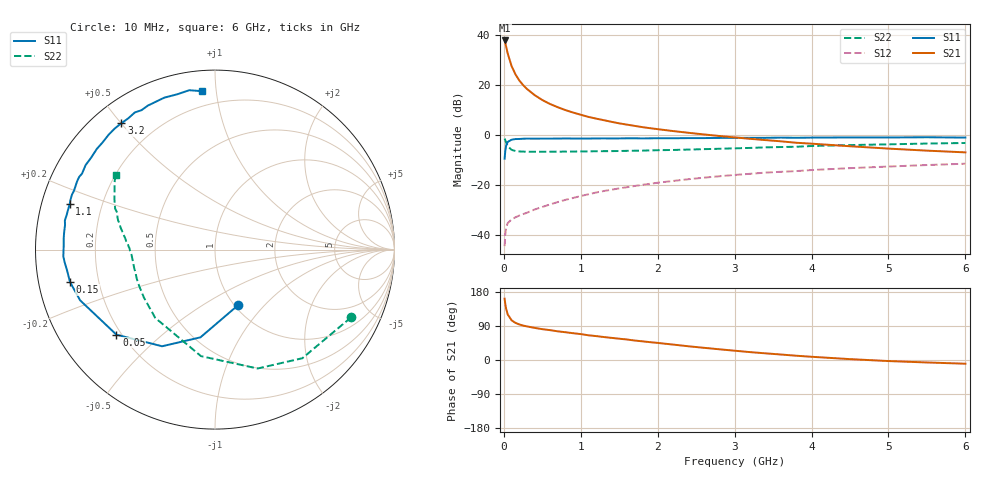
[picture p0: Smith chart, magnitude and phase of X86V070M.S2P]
! SIEMENS Small Signal Semiconductors
! BFP136W
! Si NPN RF Bipolar Junction Transistor in SOT343
! VCE = 6 V  IC = 70 mA
! Common Emitter S-Parameters:  September  1994
# GHz  S  MA  R  50
!  f  S11  S21  S12  S22
! GHz  MAG  ANG  MAG  ANG  MAG  ANG  MAG  ANG
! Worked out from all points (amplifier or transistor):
!   40 points, 10 MHz to 6 GHz, reference 50 ohm
!   highest |S21| = 37.8 dB at 10 MHz (marker M1)
!   |S21| within 3 dB of that: start of sweep to 34.05 MHz
!   unconditionally stable (mu >= 1): 612.6 MHz to 2.891 GHz
!   at 200 MHz: K = 0.59, MSG = 27.0 dB, |S12| = -32.2 dB
!   at 1.5 GHz: K = 1.10, MAG = 11.0 dB, |S12| = -21.4 dB
!   at 6 GHz: K = 0.95, MSG = 2.3 dB, |S12| = -11.5 dB
!   S11 on the Smith chart (normalised r, x): 10 MHz: 1.04, -0.72; 50 MHz: 0.18, -0.36; 150 MHz: 0.10, -0.11; 1.1 GHz: 0.08, +0.15; 3.2 GHz: 0.08, +0.50; 6 GHz: 0.11, +0.91
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0.01  0.3356 -67.6  77.28 161.8  0.006 69.4  0.8468 -26.5
0.02  0.4954 -99.4  67.65 146.4  0.0107 60.4  0.7766 -51.2
0.03  0.614 -118.7  58.31 135.0  0.0142 51.5  0.7037 -70.3
0.05  0.7254 -139.2  42.57 120.4  0.0173 39.8  0.5986 -97.5
0.1  0.8029 -159.4  23.95 104.9  0.0205 33.7  0.5055 -131.2
0.15  0.8278 -167.4  16.35 98.1  0.0226 35.0  0.4778 -146.0
0.2  0.8319 -171.8  12.31 93.9  0.0245 36.8  0.4687 -154.2
0.25  0.841 -175.3  9.939 90.9  0.0262 39.2  0.4652 -159.4
0.3  0.8459 -177.5  8.313 88.7  0.0279 41.8  0.462 -162.9
0.4  0.8432 178.4  6.258 84.7  0.0324 46.5  0.4618 -167.6
0.5  0.8454 175.6  4.99 81.4  0.0364 49.9  0.4617 -170.6
0.6  0.8459 173.3  4.161 78.8  0.0409 52.2  0.4625 -172.6
0.7  0.8467 170.7  3.588 75.7  0.0456 54.8  0.4637 -174.0
0.9  0.8486 166.8  2.806 70.7  0.0551 56.9  0.4663 -176.7
1.1  0.8483 162.5  2.294 65.2  0.0653 58.2  0.4705 -178.3
1.5  0.8533 155.8  1.706 56.2  0.0856 58.2  0.4781 178.7
1.8  0.8532 150.3  1.435 49.3  0.1008 56.7  0.4866 176.4
2.2  0.8594 143.4  1.196 40.7  0.1205 54.2  0.5012 173.5
3.2  0.8762 126.5  0.838 20.8  0.1674 45.6  0.5508 164.9
4.5  0.8924 108.5  0.595 2.3  0.2172 34.0  0.628 153.2
5.5  0.8995 99.2  0.486 -6.5  0.2506 26.0  0.6737 146.2
6  0.886 94.8  0.449 -9.8  0.2667 21.7  0.6911 143.2
